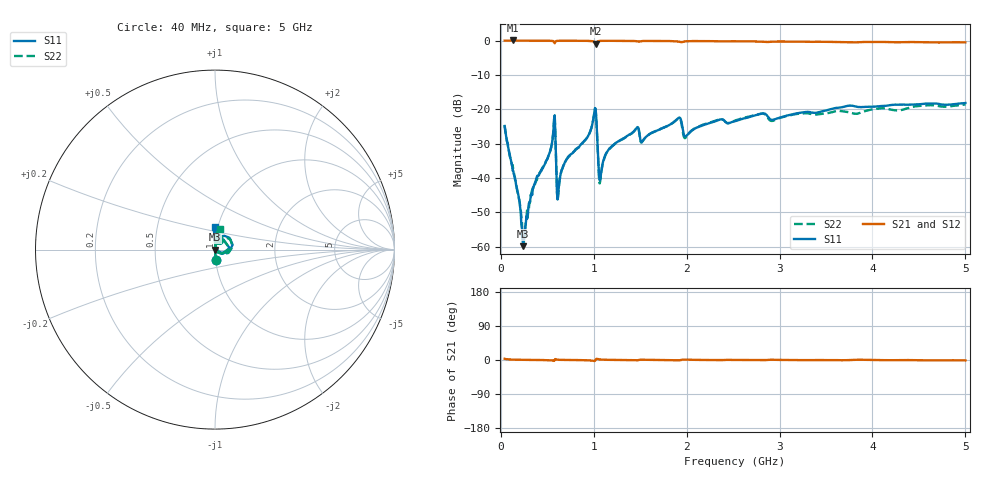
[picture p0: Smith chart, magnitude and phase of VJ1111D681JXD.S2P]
! VJ1111D681JXD
! DATE 02/15/2022  13:49
! CAPACITORS MOUNTED IN SERIES ON 25 MIL THICK MICROSTRIP SUBSTRATE
# GHz  S  MA  R  50.00
!  FREQ  S11M  S11A  S21M  S21A  S12M  S12A  S22M  S22A
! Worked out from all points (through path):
!   801 points, 40 MHz to 5 GHz, reference 50 ohm
!   highest |S21| = 0.04 dB at 126.8 MHz (marker M1); lowest = -0.9 dB at 1.02 GHz (marker M2)
!   lowest |S11| = -59.9 dB at 238.4 MHz (marker M3), VSWR 1.00, Z = 50.1 - j0.0437 ohm
!   |S11| at or under -10 dB: start of sweep to end of sweep
!   |S22| runs from -59.6 to -18.6 dB; largest |S21 - S12| = 0.011
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0.04  0.0571 -83.4  0.9986 3.2  0.998 3.4  0.05863 -84.4
0.1268  0.01275 -89.0  1.004 1.3  0.9991 1.0  0.01547 -79.7
0.2384  0.001017 -25.4  0.9987 0.4  0.9983 0.4  0.001227 -34.7
0.3686  0.008631 83.4  0.9953 0.1  1.001 0.0  0.008232 77.2
0.5112  0.02083 83.8  0.9947 -0.4  0.9988 -0.2  0.02085 82.3
0.5608  0.04205 75.5  0.986 -1.5  0.9907 -1.3  0.04184 74.2
0.6228  0.007266 69.3  0.9921 0.5  0.9997 0.6  0.007151 65.7
0.6972  0.01767 85.6  0.9953 0.1  0.9984 0.1  0.01768 82.9
0.8708  0.03165 87.1  0.9927 -0.4  0.9981 -0.4  0.03131 83.1
1.001  0.08144 65.6  0.961 -2.6  0.9637 -2.7  0.07983 59.7
1.0196  0.1017 15.2  0.8983 0.5  0.9007 0.4  0.09933 8.8
1.0568  0.0112 0.6  0.9862 1.7  0.989 1.7  0.009443 -4.1
1.0754  0.01089 60.8  0.9909 1.2  0.9941 1.1  0.01064 59.9
1.1374  0.02346 86.5  0.993 0.5  0.9967 0.5  0.02311 82.6
1.2428  0.03276 88.9  0.992 0.2  0.9969 0.1  0.03262 83.9
1.6954  0.05001 90.6  0.9873 -0.1  0.9929 -0.2  0.05007 82.5
1.9124  0.07496 75.9  0.9653 -1.0  0.9704 -1.0  0.07385 65.8
1.993  0.04046 76.7  0.9769 1.1  0.9825 1.1  0.03922 70.8
2.52  0.06734 90.6  0.9774 0.1  0.9839 -0.0  0.06841 82.2
3.3508  0.08966 88.6  0.9593 -0.0  0.9638 -0.2  0.08455 78.2
4.1754  0.1142 88.5  0.9507 -0.5  0.9589 -0.7  0.1003 77.9
5  0.1233 88.9  0.9427 -1.0  0.9487 -1.3  0.1174 76.6
